| TEXAS INSTRUMENTS INCORPORATED
| Standard Linear and Logic Group
| IBIS Model of SN74LV541AT
| Octal Buffer/Driver With 3-State Outputs
| This file contains package information for the following:
|  SOIC 20-pin (DW) package as [Component] LV541AT_DW
|  SOP 20-pin (NS) package as [Component] LV541AT_NS
|  SSOP 20-pin (DB) package as [Component] LV541AT_DB
|  TSSOP 20-pin (PW) package as [Component] LV541AT_PW
|  TVSOP 20-pin (DGV) package as [Component] LV541AT_DGV
|  QFN 20-pin (RGY) package as [Component] LV541AT_RGY
| This device can be powered at the following Vccs:
|  5 volt Vcc
| This file provides unique models under the [Model Selector] for each Vcc.
| For operation at a specific Vcc, select the appropriate model after each
| [Model Selector] keyword.
[IBIS Ver]   3.2
[Comment char]  |_char
[File Name]   sn74lv541at.ibs
[File Rev]   2.1 | x_die
[Date]   June 15, 2003
[Source]   Data created from TI-SPICE simulations at TI-SLL.
[Notes]   The following is an IBIS list for the LV541AT.
   Please contact sllibis@ti.com with questions and
   comments concerning SLL IBIS models.
   - FILE REV HISTORY
   - 2.1 Release IBIS file on 06/17/04
   - Non-monotonice data in pullup due to Ioff circuitry at output.
   - Power clamp data deleted as there is no power-clamp diode.
[Disclaimer] Property of Texas Instruments Incorporated.  Unauthorized
   reproduction and/or distribution is strictly prohibited.
   This product is protected under copyright law.
   Created  2003, (C) Copyright  2003, Texas Instruments
   Incorporated, All Rights Reserved
   UNLESS THERE IS A SIGNED, WRITTEN AGREEMENT TO THE
   CONTRARY, TEXAS INSTRUMENTS (TI) IS PROVIDING THE IBIS
   MODELS  AND WITHOUT ANY WARRANTY, EXPRESSED OR
   IMPLIED.  TI assumes no liability for:
   1) the accuracy of the IBIS models provided to your
   company;
   2) the proper functioning of these IBIS Models in your
   design or for any resulting applications; or
   3) infringement of patents, copyrights or intellectual
   property rights resulting from your use of these IBIS
   models.
   TI provides IBIS Models as a service to our customers.
   You and your company shall not distribute, sell or give
   these models to anyone else without prior written
   permission from TI.
   TI reserves the right to make changes to our products or
   to discontinue any semiconductor product or service
   without notice, and advises our customers to obtain the
   latest version of relevant information to verify, before
   placing orders, that the information being relied on is
   current.
   Please be aware that your receipt and use of the IBIS
   information provided shall serve as acceptance of these
   terms and conditions.  If you do not accept these terms,
   you should return or destroy the IBIS models and any
   other accompanying information immediately.
| Component LV541AT_DW 20-pin SOIC
[Component]   LV541AT_DW
[Manufacturer]   Texas Instruments, Inc.
[Package]
|   typ   min   max
R_pkg   3.800e-02   3.300e-02   4.500e-02
L_pkg   5.012e-09   4.110e-09   6.349e-09
C_pkg   7.170e-13   5.300e-13   8.680e-13
[Pin]   signal_name   model_name   R_pin   L_pin   C_pin
1   NOE1   LV541AT_IN   4.200e-02   6.336e-09   8.650e-13
2   A1   LV541AT_IN   4.300e-02   5.542e-09   8.670e-13
3   A2   LV541AT_IN   3.400e-02   4.714e-09   7.320e-13
4   A3   LV541AT_IN   3.400e-02   4.377e-09   5.910e-13
5   A4   LV541AT_IN   3.600e-02   4.130e-09   5.330e-13
6   A5   LV541AT_IN   3.500e-02   4.111e-09   5.300e-13
7   A6   LV541AT_IN   3.400e-02   4.284e-09   5.830e-13
8   A7   LV541AT_IN   3.400e-02   4.634e-09   7.260e-13
9   A8   LV541AT_IN   4.000e-02   5.518e-09   8.650e-13
10   GND   GND   4.300e-02   6.349e-09   8.660e-13
11   Y8   LV541AT_OUT   4.100e-02   6.281e-09   8.610e-13
12   Y7   LV541AT_OUT   4.500e-02   5.561e-09   8.680e-13
13   Y6   LV541AT_OUT   3.300e-02   4.778e-09   7.420e-13
14   Y5   LV541AT_OUT   3.500e-02   4.414e-09   5.960e-13
15   Y4   LV541AT_OUT   3.500e-02   4.110e-09   5.330e-13
16   Y3   LV541AT_OUT   3.600e-02   4.130e-09   5.330e-13
17   Y2   LV541AT_OUT   3.400e-02   4.377e-09   5.910e-13
18   Y1   LV541AT_OUT   3.400e-02   4.714e-09   7.310e-13
19   NOE2   LV541AT_IN   4.300e-02   5.569e-09   8.680e-13
20   VCC   POWER   4.200e-02   6.308e-09   8.640e-13
| Component LV541AT_NS 20-pin SOP
[Component]   LV541AT_NS
[Manufacturer]   Texas Instruments, Inc.
[Package]
|   typ   min   max
R_pkg   4.400e-02   2.900e-02   5.800e-02
L_pkg   3.666e-09   2.317e-09   5.115e-09
C_pkg   5.480e-13   3.160e-13   7.250e-13
[Pin]   signal_name   model_name   R_pin   L_pin   C_pin
1   NOE1   LV541AT_IN   5.800e-02   5.115e-09   7.250e-13
2   A1   LV541AT_IN   5.300e-02   4.591e-09   7.240e-13
3   A2   LV541AT_IN   4.900e-02   3.754e-09   5.720e-13
4   A3   LV541AT_IN   2.900e-02   2.549e-09   3.880e-13
5   A4   LV541AT_IN   3.100e-02   2.317e-09   3.160e-13
6   A5   LV541AT_IN   3.100e-02   2.317e-09   3.160e-13
7   A6   LV541AT_IN   2.900e-02   2.556e-09   3.990e-13
8   A7   LV541AT_IN   4.900e-02   3.754e-09   5.790e-13
9   A8   LV541AT_IN   5.300e-02   4.591e-09   7.240e-13
10   GND   GND   5.800e-02   5.115e-09   7.250e-13
11   Y8   LV541AT_OUT   5.800e-02   5.115e-09   7.250e-13
12   Y7   LV541AT_OUT   5.300e-02   4.591e-09   7.240e-13
13   Y6   LV541AT_OUT   4.900e-02   3.754e-09   5.790e-13
14   Y5   LV541AT_OUT   2.900e-02   2.557e-09   3.990e-13
15   Y4   LV541AT_OUT   3.100e-02   2.317e-09   3.160e-13
16   Y3   LV541AT_OUT   3.100e-02   2.317e-09   3.160e-13
17   Y2   LV541AT_OUT   2.900e-02   2.557e-09   3.990e-13
18   Y1   LV541AT_OUT   4.900e-02   3.754e-09   5.790e-13
19   NOE2   LV541AT_IN   5.300e-02   4.591e-09   7.240e-13
20   VCC   POWER   5.800e-02   5.115e-09   7.250e-13
| Component LV541AT_DB 20-pin SSOP
[Component]   LV541AT_DB
[Manufacturer]   Texas Instruments, Inc.
[Package]
|   typ   min   max
R_pkg   4.000e-02   3.500e-02   5.100e-02
L_pkg   3.495e-09   3.035e-09   4.314e-09
C_pkg   4.200e-13   3.460e-13   5.020e-13
[Pin]   signal_name   model_name   R_pin   L_pin   C_pin
1   NOE1   LV541AT_IN   4.900e-02   4.310e-09   5.020e-13
2   A1   LV541AT_IN   4.800e-02   3.903e-09   4.870e-13
3   A2   LV541AT_IN   3.500e-02   3.189e-09   3.960e-13
4   A3   LV541AT_IN   3.500e-02   3.036e-09   3.470e-13
5   A4   LV541AT_IN   3.500e-02   3.035e-09   3.670e-13
6   A5   LV541AT_IN   3.500e-02   3.035e-09   3.670e-13
7   A6   LV541AT_IN   3.500e-02   3.036e-09   3.470e-13
8   A7   LV541AT_IN   3.500e-02   3.189e-09   3.970e-13
9   A8   LV541AT_IN   4.700e-02   3.899e-09   4.880e-13
10   GND   GND   5.100e-02   4.314e-09   5.000e-13
11   Y8   LV541AT_OUT   5.100e-02   4.314e-09   5.000e-13
12   Y7   LV541AT_OUT   4.700e-02   3.899e-09   4.880e-13
13   Y6   LV541AT_OUT   3.500e-02   3.189e-09   3.970e-13
14   Y5   LV541AT_OUT   3.500e-02   3.036e-09   3.460e-13
15   Y4   LV541AT_OUT   3.500e-02   3.035e-09   3.670e-13
16   Y3   LV541AT_OUT   3.500e-02   3.035e-09   3.670e-13
17   Y2   LV541AT_OUT   3.500e-02   3.036e-09   3.460e-13
18   Y1   LV541AT_OUT   3.500e-02   3.189e-09   3.970e-13
19   NOE2   LV541AT_IN   4.700e-02   3.899e-09   4.880e-13
20   VCC   POWER   5.100e-02   4.314e-09   5.020e-13
| Component LV541AT_PW 20-pin TSSOP
[Component]   LV541AT_PW
[Manufacturer]   Texas Instruments, Inc.
[Package]
|   typ   min   max
R_pkg   5.000e-02   4.200e-02   6.000e-02
L_pkg   2.802e-09   2.248e-09   3.553e-09
C_pkg   3.170e-13   2.020e-13   4.430e-13
[Pin]   signal_name   model_name   R_pin   L_pin   C_pin
1   NOE1   LV541AT_IN   5.500e-02   3.461e-09   4.400e-13
2   A1   LV541AT_IN   5.500e-02   3.150e-09   4.010e-13
3   A2   LV541AT_IN   4.200e-02   2.619e-09   3.020e-13
4   A3   LV541AT_IN   4.500e-02   2.273e-09   2.020e-13
5   A4   LV541AT_IN   4.500e-02   2.248e-09   2.240e-13
6   A5   LV541AT_IN   4.500e-02   2.273e-09   2.260e-13
7   A6   LV541AT_IN   4.400e-02   2.323e-09   2.050e-13
8   A7   LV541AT_IN   4.600e-02   2.704e-09   3.070e-13
9   A8   LV541AT_IN   6.000e-02   3.265e-09   4.110e-13
10   GND   GND   5.700e-02   3.506e-09   4.360e-13
11   Y8   LV541AT_OUT   5.800e-02   3.553e-09   4.370e-13
12   Y7   LV541AT_OUT   5.800e-02   3.193e-09   4.050e-13
13   Y6   LV541AT_OUT   4.200e-02   2.704e-09   3.110e-13
14   Y5   LV541AT_OUT   4.600e-02   2.392e-09   2.100e-13
15   Y4   LV541AT_OUT   4.700e-02   2.334e-09   2.290e-13
16   Y3   LV541AT_OUT   4.700e-02   2.300e-09   2.270e-13
17   Y2   LV541AT_OUT   4.700e-02   2.349e-09   2.070e-13
18   Y1   LV541AT_OUT   4.500e-02   2.677e-09   3.060e-13
19   NOE2   LV541AT_IN   6.000e-02   3.235e-09   4.060e-13
20   VCC   POWER   5.600e-02   3.487e-09   4.430e-13
| Component LV541AT_DGV 20-pin TVSOP
[Component]   LV541AT_DGV
[Manufacturer]   Texas Instruments, Inc.
[Package]
|   typ   min   max
R_pkg   4.400e-02   3.800e-02   4.800e-02
L_pkg   2.561e-09   2.236e-09   2.961e-09
C_pkg   3.420e-13   2.640e-13   4.460e-13
[Pin]   signal_name   model_name   R_pin   L_pin   C_pin
1   NOE1   LV541AT_IN   4.400e-02   2.935e-09   4.170e-13
2   A1   LV541AT_IN   4.200e-02   2.869e-09   4.460e-13
3   A2   LV541AT_IN   4.300e-02   2.399e-09   3.160e-13
4   A3   LV541AT_IN   4.400e-02   2.236e-09   2.650e-13
5   A4   LV541AT_IN   4.600e-02   2.278e-09   2.640e-13
6   A5   LV541AT_IN   4.500e-02   2.274e-09   2.640e-13
7   A6   LV541AT_IN   4.400e-02   2.285e-09   2.690e-13
8   A7   LV541AT_IN   4.300e-02   2.452e-09   3.200e-13
9   A8   LV541AT_IN   4.400e-02   2.900e-09   4.460e-13
10   GND   GND   4.400e-02   2.961e-09   4.180e-13
11   Y8   LV541AT_OUT   4.500e-02   2.954e-09   4.180e-13
12   Y7   LV541AT_OUT   4.200e-02   2.847e-09   4.430e-13
13   Y6   LV541AT_OUT   4.500e-02   2.453e-09   3.190e-13
14   Y5   LV541AT_OUT   4.500e-02   2.297e-09   2.690e-13
15   Y4   LV541AT_OUT   4.800e-02   2.334e-09   2.680e-13
16   Y3   LV541AT_OUT   4.800e-02   2.335e-09   2.670e-13
17   Y2   LV541AT_OUT   4.600e-02   2.299e-09   2.680e-13
18   Y1   LV541AT_OUT   4.600e-02   2.457e-09   3.200e-13
19   NOE2   LV541AT_IN   4.300e-02   2.848e-09   4.410e-13
20   VCC   POWER   3.800e-02   2.812e-09   4.080e-13
| Component LV541AT_RGY 20-pin QFN
[Component]   LV541AT_RGY
[Manufacturer]   Texas Instruments, Inc.
[Package]
|   typ   min   max
R_pkg   0.046   0.035   0.058
L_pkg   1.131nH   0.880nH   1.396nH
C_pkg   0.165pF   0.142pF   0.175pF
[Pin]   signal_name   model_name   R_pin   L_pin   C_pin
1   NOE1   LV541AT_IN   0.053   1.289nH   0.142pF
2   A1   LV541AT_IN   0.058   1.386nH   0.172pF
3   A2   LV541AT_IN   0.046   1.111nH   0.173pF
4   A3   LV541AT_IN   0.039   0.965nH   0.161pF
5   A4   LV541AT_IN   0.035   0.881nH   0.165pF
6   A5   LV541AT_IN   0.035   0.880nH   0.165pF
7   A6   LV541AT_IN   0.039   0.961nH   0.161pF
8   A7   LV541AT_IN   0.045   1.105nH   0.172pF
9   A8   LV541AT_IN   0.058   1.386nH   0.172pF
10   GND   GND   0.056   1.352nH   0.159pF
11   Y8   LV541AT_OUT   0.053   1.287nH   0.155pF
12   Y7   LV541AT_OUT   0.058   1.396nH   0.172pF
13   Y6   LV541AT_OUT   0.047   1.129nH   0.175pF
14   Y5   LV541AT_OUT   0.040   0.976nH   0.164pF
15   Y4   LV541AT_OUT   0.035   0.884nH   0.169pF
16   Y3   LV541AT_OUT   0.035   0.881nH   0.168pF
17   Y2   LV541AT_OUT   0.039   0.967nH   0.162pF
18   Y1   LV541AT_OUT   0.046   1.118nH   0.174pF
19   NOE2   LV541AT_IN   0.058   1.396nH   0.175pF
20   VCC   POWER   0.052   1.276nH   0.144pF
| Models and submodels in the file (2): LV541AT_IN (Input), LV541AT_OUT (3-state)
